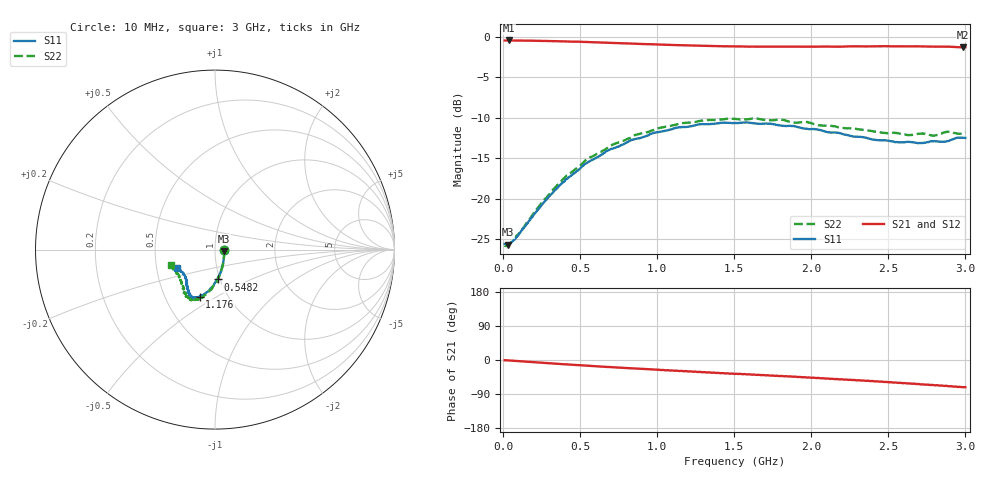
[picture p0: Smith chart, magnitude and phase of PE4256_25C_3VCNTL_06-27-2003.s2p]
!Peregrine Semiconductor Corp.
!S-Parameter Data for Device PE4256 in IL PATH with TEMP = 25C
!File Created On: 06-27-2003
!Start Frequency = 1.000E+01
!Stop Frequency = 3.000E+03
!Number of Points = 401
# MHZ S DB R 75
!Freq  S11MAG  S11PH  S12MAG  S12PH  S21MAG  S21PH  S22MAG  S22PH
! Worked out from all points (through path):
!   401 points, 10 MHz to 3 GHz, reference 75 ohm
!   highest |S21| = -0.48 dB at 39.9 MHz (marker M1); lowest = -1.3 dB at 2.985 GHz (marker M2)
!   group delay of S21, straight-line fit = 63.2 ps
!   lowest |S11| = -25.7 dB at 32.43 MHz (marker M3), VSWR 1.11, Z = 83 - j1.68 ohm
!   |S11| at or under -10 dB: start of sweep to end of sweep
!   |S22| runs from -25.9 to -10.1 dB; largest |S21 - S12| = 0.0055
!   S11 on the Smith chart (normalised r, x): 10 MHz: 1.11, -0.01; 548.2 MHz: 0.97, -0.33; 1.176 GHz: 0.74, -0.42; 3 GHz: 0.64, -0.14
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10  -25.60 -4.9  -0.49 -0.6  -0.47 -0.5  -25.79 -5.2
32.43  -25.70 -11.2  -0.48 -1.0  -0.46 -1.1  -25.76 -11.8
39.9  -25.54 -13.7  -0.48 -1.3  -0.47 -1.3  -25.60 -14.6
84.75  -24.79 -28.3  -0.48 -2.5  -0.48 -2.5  -24.66 -29.5
323.95  -19.25 -69.3  -0.56 -9.4  -0.56 -9.4  -18.87 -70.3
398.7  -17.88 -75.6  -0.60 -11.3  -0.59 -11.3  -17.45 -76.7
510.83  -16.06 -83.8  -0.65 -14.2  -0.64 -14.2  -15.77 -84.2
548.2  -15.55 -85.2  -0.68 -15.0  -0.67 -15.0  -15.11 -86.2
705.18  -13.86 -92.7  -0.78 -18.9  -0.78 -18.9  -13.41 -94.0
824.78  -12.83 -97.8  -0.86 -21.7  -0.86 -21.7  -12.52 -98.6
1011.65  -11.78 -103.3  -0.98 -25.8  -0.98 -25.8  -11.29 -104.3
1176.1  -11.16 -108.0  -1.08 -29.7  -1.08 -29.7  -10.66 -109.0
1505  -10.68 -115.8  -1.21 -36.8  -1.20 -36.7  -10.16 -116.2
1721.77  -10.77 -119.6  -1.24 -40.5  -1.23 -40.5  -10.34 -120.0
2005.82  -11.42 -125.2  -1.26 -47.1  -1.23 -47.1  -10.73 -125.9
2506.65  -12.88 -136.6  -1.20 -58.9  -1.19 -58.9  -11.91 -141.7
2633.72  -13.00 -140.9  -1.21 -61.6  -1.19 -61.6  -12.17 -145.2
2708.47  -13.15 -143.5  -1.21 -64.0  -1.21 -64.0  -11.97 -148.6
2798.17  -12.92 -147.2  -1.25 -66.5  -1.22 -66.4  -12.22 -151.8
2887.87  -12.90 -150.7  -1.25 -68.9  -1.25 -68.9  -11.76 -155.1
2985.05  -12.50 -154.0  -1.33 -72.0  -1.29 -71.9  -11.90 -160.2
3000  -12.51 -154.1  -1.32 -71.9  -1.30 -71.9  -11.77 -160.8
